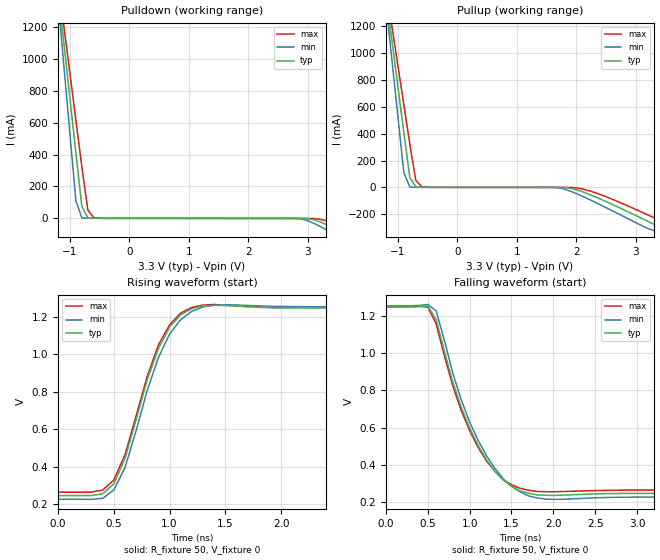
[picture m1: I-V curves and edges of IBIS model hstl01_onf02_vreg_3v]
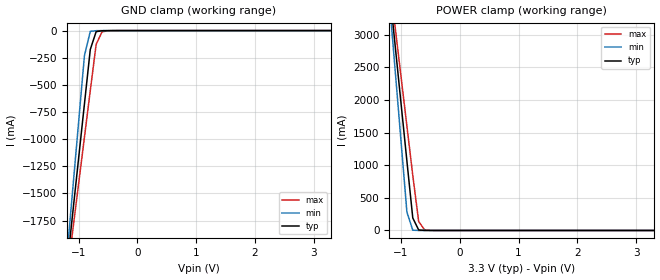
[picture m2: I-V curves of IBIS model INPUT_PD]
|   This file is an IBIS representation of the   |
|   Integrated Device Technology, Inc.   |
|   ICS85222-01   |
|   Dual LVCMOS/LVTTL-to-Differential HSTL Translator   |
[IBIS Ver]   4.0
[File name]   85222-01_3v3.ibs
[File Rev]   1.0
[Date]   Jun 5 2006 | Last modified
|   Jun 5 2006 | Generated
[Source] Originated at Integrated Device Technology, Inc.
[Disclaimer]
IDT hereby grants the user of this IBIS model a non-exclusive,
nontransferable license to use this IBIS model under the following terms.
Before using this IBIS model, the user should read this license.
If the user does not accept these terms,  the IBIS model should be
returned to IDT within 30 days.
   The user is granted this license only to use the IBIS model and
is not granted rights to sell, load, rent, lease or license the IBIS
model in whole or in part, or in modified form to anyone other than
user. User may modify the IBIS model to suit its specific
applications but rights to derivative works and such modifications
shall belong to ICS.
   This IBIS model is provided on an "AS IS" basis and IDT makes
absolutely no warranty with respect to the information contained
herein. IDT DISCLAIMS AND CUSTOMER WAIVES ALL WARRANTIES, EXPRESS
OR IMPLIED, INCLUDING WARRANTIES OF MERCHANTABILITY OR FITNESS FOR
A PARTICULAR PURPOSE. The entire risk as to quality and performance
is with the Customer. ACCORDINGLY, IN NO EVENT SHALL THE COMPANY BE
LIABLE FOR ANY DAMAGES, WHETHER IN CONTRACT OR TORT,INCLUDING ANY
LOST PROFITS OR OTHER INCIDENTAL, CONSEQUENTIAL, EXEMPLARY, OR
PUNITIVE DAMAGES ARISING OUT OF THE USE OR APPLICATION OF THE IBIS
model provided in this package. Further, IDT reserves the right to
make changes without notice to any product herein to improve
reliability, function, or design. IDT does not convey any license
under patent rights or any other intellectual property rights,
including those of third parties.
   IDT is not obligated to provide maintenance or support
for the licensed IBIS model.
[Copyright]   Copyright 2006 by Integrated Device Technology, Inc.
[Component]   ICS85222AM-01
[Manufacturer] Integrated Device Technology, Inc.
[Package]
|SOIC 8 Lead
|   typ   min   max
R_pkg   57.05m   55.5m   58.6m
L_pkg   1.769nH   1.570nH   1.968nH
C_pkg   0.269pF   0.252pF   0.286pF
[Pin] signal_name   model_name
1   Q0   hstl01_onf02_vreg_3v
2   nQ0   hstl01_onf02_vreg_3v
3   Q1   hstl01_onf02_vreg_3v
4   nQ1   hstl01_onf02_vreg_3v
5   GND   GND
6   CLK1   INPUT_PD
7   CLK0   INPUT_PD
8   VDD   Power
[Diff Pin]  inv_pin  vdiff tdelay_typ tdelay_min  tdelay_max
1   2   NA   0  0  0
3   4   NA   0  0  0
| Models and submodels in the file (2): hstl01_onf02_vreg_3v (Output_ECL), INPUT_PD (Input)
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[Model]   hstl01_onf02_vreg_3v
Model_type  Output_ECL
Polarity   Non-Inverting
Vmeas = 0.7
Rref = 50
Cref = 0
Vref = 0
|Variable   typ   min   max
C_comp   2p   1.5p   2.5p
[Voltage Range]   3.3V   3.135V   3.465V
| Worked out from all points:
|   rising waveform, R_fixture 50, V_fixture 0: 20-80 % time 313ps typ, 334ps min, 304ps max; typ from 0.247 V to 1.25 V
|   falling waveform, R_fixture 50, V_fixture 0: 20-80 % time 500ps typ, 517ps min, 486ps max; typ from 1.25 V to 0.247 V
|  Voltage   I(typ)   I(min)   I(max)
[Pullup]
-3.3V     8.641A     10.21A     7.646A
-1.2V     1.434A     1.367A     1.49A
-1.1V     1.093A     948mA      1.198A
-1V       751.3mA    529.2mA    906.5mA
-900mV    410.6mA    111.1mA    615.5mA
-800mV    75.74mA    3.773mA    324.8mA
-700mV    4.471mA    906.8uA    54.01mA
-600mV    1.036mA    546.9uA    4.666mA
1.7V      185.8uA    -2.662mA   271.8uA
1.9V      -6.371mA   -28.06mA   -89.47uA
2.2V      -48.56mA   -85.92mA   -22.7mA
3.3V      -273.4mA   -320.7mA   -224.7mA
[Pulldown]
-3.3V     8.641A     10.21A     7.646A
-1.2V     1.434A     1.367A     1.49A
-1.1V     1.093A     948mA      1.198A
-1V       751.3mA    529.2mA    906.5mA
-900mV    410.6mA    111.1mA    615.5mA
-800mV    75.74mA    3.773mA    324.8mA
-700mV    4.471mA    906.8uA    54.01mA
-600mV    1.036mA    546.9uA    4.666mA
2.8V      -101uA     -377.4uA   -71.09uA
2.9V      -231.6uA   -3.941mA   -95.27uA
3.1V      -9.095mA   -30.96mA   -946uA
3.3V      -36.64mA   -68.55mA   -14.52mA
[Ramp]
|   typ   min   max
dV/dt_r   0.6V/0.55ns   0.6V/0.65ns   0.6V/0.45ns
dV/dt_f   0.6V/0.3ns   0.6V/0.35ns   0.6V/0.25ns
R_load =   50.0000
[Rising Waveform]
R_fixture = 50
V_fixture = 0
C_fixture = 0.0p
| Time   typ   min   max
0s        247mV      227.2mV    264.7mV
400ps     256.2mV    232mV      276.3mV
500ps     309.7mV    277mV      329.8mV
600ps     444.5mV    395.9mV    463.9mV
800ps     865.6mV    807.8mV    883mV
900ps     1.03V      982.1mV    1.049V
1ns       1.144V     1.107V     1.156V
1.2ns     1.243V     1.228V     1.249V
1.5ns     1.259V     1.262V     1.261V
4ns       1.246V     1.253V     1.248V
[Falling Waveform]
R_fixture = 50
V_fixture = 0
C_fixture = 0.0p
| Time   typ   min   max
0s        1.247V     1.253V     1.248V
500ps     1.251V     1.26V      1.246V
600ps     1.179V     1.226V     1.156V
800ps     841.3mV    889.9mV    821.8mV
900ps     708.2mV    747.8mV    690.9mV
1.1ns     504.5mV    531.8mV    494.4mV
1.4ns     318.8mV    326.1mV    320.5mV
1.6ns     259.5mV    255.1mV    274.2mV
2ns       235.6mV    214.7mV    255.1mV
4ns       246.7mV    226.8mV    264.4mV
[Model]   INPUT_PD
Model_type   Input
Polarity   Non-Inverting
Vinl = 1.4V
Vinh = 1.85V
|   typ   min   max
C_comp   2pF   1.5pF   2.5pF
|   typ   min   max
[Voltage range]  3.3V   3.15V   3.45V
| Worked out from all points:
|   GND clamp passes 1 mA (typ) near -0.55 V on its own axis
|   POWER clamp passes 1 mA (typ) near -0.60 V on its own axis
[GND_clamp]
|Voltage I(typ)   I(min)   I(max)
-3.3V     -12.83A    -15.14A    -11.37A
-1.2V     -2.195A    -2.092A    -2.281A
-1.1V     -1.689A    -1.472A    -1.849A
-900mV    -678.5mA   -232.6mA   -984.8mA
-800mV    -173.9mA   -7.175mA   -553.2mA
-700mV    -9.696mA   -1.052mA   -126mA
-600mV    -1.629mA   -178uA     -11.07mA
-300mV    -10.53uA   -5.678uA   -86.08uA
3.3V      71.13uA    62.11uA    77.58uA
[POWER_clamp]
|Voltage   I(typ)   I(min)   I(max)
-3.3V     22.38A     26.45A     19.82A
-1.2V     3.723A     3.545A     3.874A
-1.1V     2.836A     2.457A     3.116A
-1V       1.949A     1.369A     2.358A
-900mV    1.063A     281.1mA    1.601A
-800mV    191.6mA    5.074mA    844mA
-700mV    8.104mA    204.3uA    138.4mA
-600mV    678.1uA    79.74uA    10.7mA
-400mV    87.44uA    69.65uA    413.2uA
3.3V      -3.041nA   -425fA     -919.9nA
